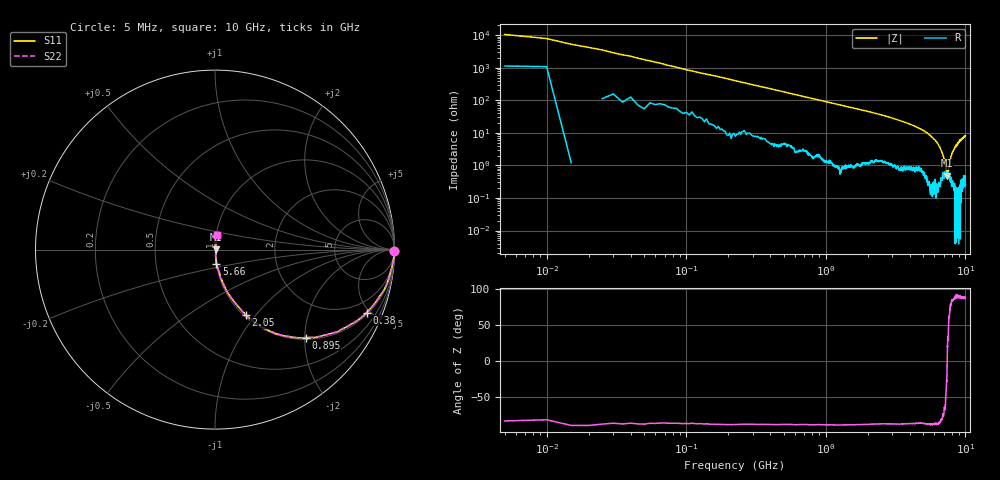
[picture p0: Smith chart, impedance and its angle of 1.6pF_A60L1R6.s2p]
! Amotech Co.,Ltd.
! http://www.amotech.co.kr/
! Part Number: A60L1R6
! These Parameters are Measured in Series Mode Connection
! Operation Temp=25[degC], DC Bias Voltage=0[V]
! Freq. Start=5[MHz] Stop=10[GHz], 2000[Steps]
! Date: Monday, July 14, 2020, 09:28:09
# GHZ S RI R 50.000000
!Freq.(Hz) S11(Real) S11(Imag) S21(Real) S21(Imag) S12(Real) S12(Imag) S22(Real) S22(Imag)
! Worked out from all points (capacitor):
!   2000 points, 5 MHz to 10 GHz, reference 50 ohm
!   read as one part in series: C = 1.81 pF near 55 MHz
!   lowest |Z| = 486 mohm at 7.425 GHz (marker M1)
!   series resonance near 7.414 GHz, so ESL is about 250 pH
!   S11 on the Smith chart (normalised r, x): 5 MHz: open; 380 MHz: 1.11, -4.77; 895 MHz: 1.04, -2.02; 2.05 GHz: 1.02, -0.89; 5.66 GHz: 1.00, -0.16; 10 GHz: 1.01, +0.16
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0.005  0.9989 -0.00947  0.00112 0.00947  0.00112 0.00947  0.9989 -0.00947
0.07  0.9893 -0.0778  0.0107 0.0778  0.0107 0.0778  0.9893 -0.0778
0.125  0.9743 -0.1378  0.0257 0.1378  0.0257 0.1378  0.9743 -0.1378
0.235  0.931 -0.2419  0.069 0.2419  0.069 0.2419  0.931 -0.2419
0.38  0.8453 -0.3506  0.1547 0.3506  0.1547 0.3506  0.8453 -0.3506
0.59  0.698 -0.448  0.302 0.448  0.302 0.448  0.698 -0.448
0.895  0.5045 -0.4905  0.4955 0.4905  0.4955 0.4905  0.5045 -0.4905
1.675  0.2323 -0.4126  0.7677 0.4126  0.7677 0.4126  0.2323 -0.4126
2.05  0.1705 -0.363  0.8295 0.363  0.8295 0.363  0.1705 -0.363
3.34  0.0618 -0.2257  0.9382 0.2257  0.9382 0.2257  0.0618 -0.2257
5.005  0.0186 -0.1147  0.9814 0.1147  0.9814 0.1147  0.0186 -0.1147
5.66  0.00808 -0.079  0.9919 0.079  0.9919 0.079  0.00808 -0.079
6.215  0.00465 -0.0533  0.9953 0.0533  0.9953 0.0533  0.00465 -0.0533
6.67  0.00467 -0.0305  0.9953 0.0305  0.9953 0.0305  0.00467 -0.0305
7.035  0.00577 -0.0148  0.9942 0.0148  0.9942 0.0148  0.00577 -0.0148
7.21  0.00586 -0.00865  0.9941 0.00865  0.9941 0.00865  0.00586 -0.00865
7.31  0.00518 -0.00368  0.9948 0.00368  0.9948 0.00368  0.00518 -0.00368
7.425  0.0048 0.000625  0.9952 -0.000625  0.9952 -0.000625  0.0048 0.000625
7.915  0.00448 0.0193  0.9955 -0.0193  0.9955 -0.0193  0.00448 0.0193
8.335  0.00314 0.0327  0.9969 -0.0327  0.9969 -0.0327  0.00314 0.0327
8.975  0.00315 0.054  0.9969 -0.054  0.9969 -0.054  0.00315 0.054
10  0.00923 0.0813  0.9908 -0.0813  0.9908 -0.0813  0.00923 0.0813
